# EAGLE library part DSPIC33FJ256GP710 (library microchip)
dsPIC33FJ256GP710_TQFP edit this description Auto generated by make-symbol-device-package-bsdl.ulp Rev. 41 Source: dsPIC33FJ256GP710_TQFP.bsd
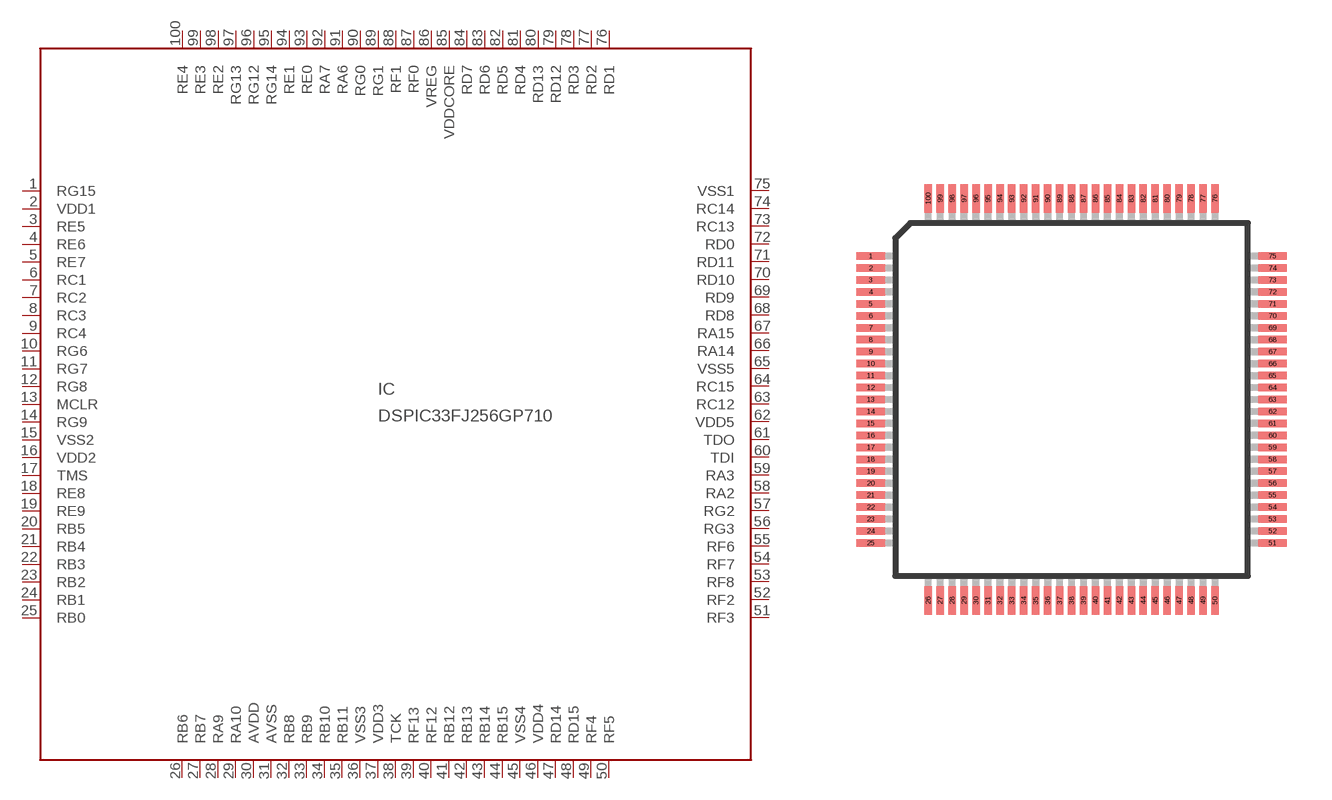
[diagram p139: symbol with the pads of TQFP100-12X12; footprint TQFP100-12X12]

Designator prefix IC

## DSPIC33FJ256GP710  [TQFP100-12X12]
1  RG15
2  VDD1  pwr
3  RE5
4  RE6
5  RE7
6  RC1
7  RC2
8  RC3
9  RC4
10  RG6
11  RG7
12  RG8
13  MCLR
14  RG9
15  VSS2  pwr
16  VDD2  pwr
17  TMS  in
18  RE8
19  RE9
20  RB5
21  RB4
22  RB3
23  RB2
24  RB1
25  RB0
26  RB6
27  RB7
28  RA9
29  RA10
30  AVDD  pwr
31  AVSS  pwr
32  RB8
33  RB9
34  RB10
35  RB11
36  VSS3  pwr
37  VDD3  pwr
38  TCK  in
39  RF13
40  RF12
41  RB12
42  RB13
43  RB14
44  RB15
45  VSS4  pwr
46  VDD4  pwr
47  RD14
48  RD15
49  RF4
50  RF5
51  RF3
52  RF2
53  RF8
54  RF7
55  RF6
56  RG3
57  RG2
58  RA2
59  RA3
60  TDI  in
61  TDO  out
62  VDD5  pwr
63  RC12
64  RC15
65  VSS5  pwr
66  RA14
67  RA15
68  RD8
69  RD9
70  RD10
71  RD11
72  RD0
73  RC13
74  RC14
75  VSS1  pwr
76  RD1
77  RD2
78  RD3
79  RD12
80  RD13
81  RD4
82  RD5
83  RD6
84  RD7
85  VDDCORE  pwr
86  VREG  pas
87  RF0
88  RF1
89  RG1
90  RG0
91  RA6
92  RA7
93  RE0
94  RE1
95  RG14
96  RG12
97  RG13
98  RE2
99  RE3
100  RE4

## Footprint TQFP100-12X12 (pad centres in mm)
TQFP100_12X12 Auto generated by make-symbol-device-package-bsdl.ulp Rev. 41
smd 0.95 x 0.25: 1 -6.725,4.8; 2 -6.725,4.4; 3 -6.725,4; 4 -6.725,3.6; 5 -6.725,3.2; 6 -6.725,2.8; 7 -6.725,2.4; 8 -6.725,2; 9 -6.725,1.6; 10 -6.725,1.2; 11 -6.725,0.8; 12 -6.725,0.4; 13 -6.725,0; 14 -6.725,-0.4; 15 -6.725,-0.8; 16 -6.725,-1.2; 17 -6.725,-1.6; 18 -6.725,-2; 19 -6.725,-2.4; 20 -6.725,-2.8; 21 -6.725,-3.2; 22 -6.725,-3.6; 23 -6.725,-4; 24 -6.725,-4.4; 25 -6.725,-4.8; 51 6.725,-4.8; 52 6.725,-4.4; 53 6.725,-4; 54 6.725,-3.6; 55 6.725,-3.2; 56 6.725,-2.8; 57 6.725,-2.4; 58 6.725,-2; 59 6.725,-1.6; 60 6.725,-1.2; 61 6.725,-0.8; 62 6.725,-0.4; 63 6.725,0; 64 6.725,0.4; 65 6.725,0.8; 66 6.725,1.2; 67 6.725,1.6; 68 6.725,2; 69 6.725,2.4; 70 6.725,2.8; 71 6.725,3.2; 72 6.725,3.6; 73 6.725,4; 74 6.725,4.4; 75 6.725,4.8
smd 0.25 x 0.95: 26 -4.8,-6.725; 27 -4.4,-6.725; 28 -4,-6.725; 29 -3.6,-6.725; 30 -3.2,-6.725; 31 -2.8,-6.725; 32 -2.4,-6.725; 33 -2,-6.725; 34 -1.6,-6.725; 35 -1.2,-6.725; 36 -0.8,-6.725; 37 -0.4,-6.725; 38 0,-6.725; 39 0.4,-6.725; 40 0.8,-6.725; 41 1.2,-6.725; 42 1.6,-6.725; 43 2,-6.725; 44 2.4,-6.725; 45 2.8,-6.725; 46 3.2,-6.725; 47 3.6,-6.725; 48 4,-6.725; 49 4.4,-6.725; 50 4.8,-6.725; 76 4.8,6.725; 77 4.4,6.725; 78 4,6.725; 79 3.6,6.725; 80 3.2,6.725; 81 2.8,6.725; 82 2.4,6.725; 83 2,6.725; 84 1.6,6.725; 85 1.2,6.725; 86 0.8,6.725; 87 0.4,6.725; 88 0,6.725; 89 -0.4,6.725; 90 -0.8,6.725; 91 -1.2,6.725; 92 -1.6,6.725; 93 -2,6.725; 94 -2.4,6.725; 95 -2.8,6.725; 96 -3.2,6.725; 97 -3.6,6.725; 98 -4,6.725; 99 -4.4,6.725; 100 -4.8,6.725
